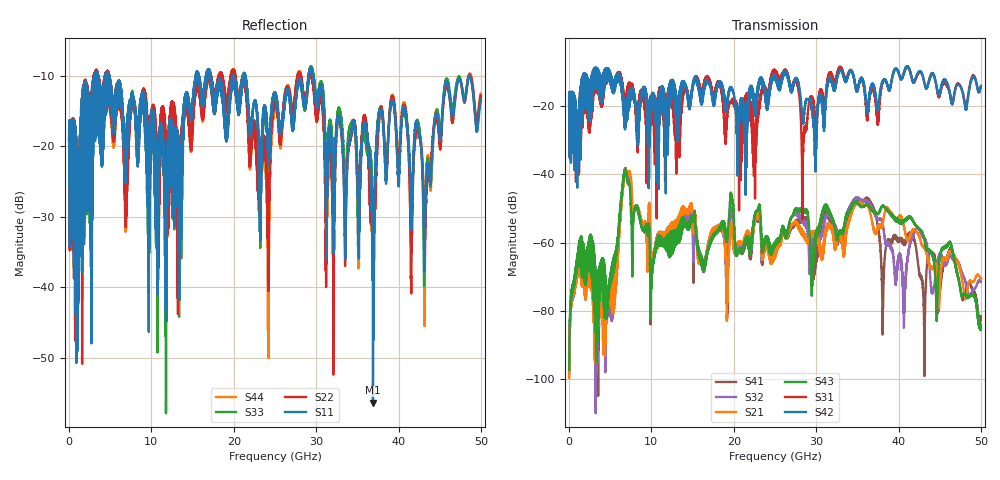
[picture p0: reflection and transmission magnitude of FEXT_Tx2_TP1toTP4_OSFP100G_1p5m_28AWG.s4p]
! Touchstone data
! Created: 27-Feb-2019 by IdEM 12 (12.1.0)
! COMMENTS
!  Created Wed Feb 27 09:43:39 2019
!  64 Port Network Data from SP1.SP block
!  freq  magS1_1  angS1_1  magS1_2  angS1_2  magS1_3  angS1_3  magS1_4  angS1_4
!  magS1_5  angS1_5  magS1_6  angS1_6  magS1_7  angS1_7  magS1_8  angS1_8
!  magS1_9  angS1_9  magS1_10  angS1_10  magS1_11  angS1_11  magS1_12  angS1_12
!  magS1_13  angS1_13  magS1_14  angS1_14  magS1_15  angS1_15  magS1_16  angS1_16
!  magS1_17  angS1_17  magS1_18  angS1_18  magS1_19  angS1_19  magS1_20  angS1_20
!  magS1_21  angS1_21  magS1_22  angS1_22  magS1_23  angS1_23  magS1_24  angS1_24
!  magS1_25  angS1_25  magS1_26  angS1_26  magS1_27  angS1_27  magS1_28  angS1_28
!  magS1_29  angS1_29  magS1_30  angS1_30  magS1_31  angS1_31  magS1_32  angS1_32
!  magS1_33  angS1_33  magS1_34  angS1_34  magS1_35  angS1_35  magS1_36  angS1_36
!  magS1_37  angS1_37  magS1_38  angS1_38  magS1_39  angS1_39  magS1_40  angS1_40
!  magS1_41  angS1_41  magS1_42  angS1_42  magS1_43  angS1_43  magS1_44  angS1_44
!  magS1_45  angS1_45  magS1_46  angS1_46  magS1_47  angS1_47  magS1_48  angS1_48
!  magS1_49  angS1_49  magS1_50  angS1_50  magS1_51  angS1_51  magS1_52  angS1_52
!  magS1_53  angS1_53  magS1_54  angS1_54  magS1_55  angS1_55  magS1_56  angS1_56
!  magS1_57  angS1_57  magS1_58  angS1_58  magS1_59  angS1_59  magS1_60  angS1_60
!  magS1_61  angS1_61  magS1_62  angS1_62  magS1_63  angS1_63  magS1_64  angS1_64
!  magS2_1  angS2_1  magS2_2  angS2_2  magS2_3  angS2_3  magS2_4  angS2_4
!  magS2_5  angS2_5  magS2_6  angS2_6  magS2_7  angS2_7  magS2_8  angS2_8
!  magS2_9  angS2_9  magS2_10  angS2_10  magS2_11  angS2_11  magS2_12  angS2_12
!  magS2_13  angS2_13  magS2_14  angS2_14  magS2_15  angS2_15  magS2_16  angS2_16
!  magS2_17  angS2_17  magS2_18  angS2_18  magS2_19  angS2_19  magS2_20  angS2_20
!  magS2_21  angS2_21  magS2_22  angS2_22  magS2_23  angS2_23  magS2_24  angS2_24
!  magS2_25  angS2_25  magS2_26  angS2_26  magS2_27  angS2_27  magS2_28  angS2_28
!  magS2_29  angS2_29  magS2_30  angS2_30  magS2_31  angS2_31  magS2_32  angS2_32
!  magS2_33  angS2_33  magS2_34  angS2_34  magS2_35  angS2_35  magS2_36  angS2_36
!  magS2_37  angS2_37  magS2_38  angS2_38  magS2_39  angS2_39  magS2_40  angS2_40
!  magS2_41  angS2_41  magS2_42  angS2_42  magS2_43  angS2_43  magS2_44  angS2_44
!  magS2_45  angS2_45  magS2_46  angS2_46  magS2_47  angS2_47  magS2_48  angS2_48
!  magS2_49  angS2_49  magS2_50  angS2_50  magS2_51  angS2_51  magS2_52  angS2_52
!  magS2_53  angS2_53  magS2_54  angS2_54  magS2_55  angS2_55  magS2_56  angS2_56
!  magS2_57  angS2_57  magS2_58  angS2_58  magS2_59  angS2_59  magS2_60  angS2_60
!  magS2_61  angS2_61  magS2_62  angS2_62  magS2_63  angS2_63  magS2_64  angS2_64
!  magS3_1  angS3_1  magS3_2  angS3_2  magS3_3  angS3_3  magS3_4  angS3_4
!  magS3_5  angS3_5  magS3_6  angS3_6  magS3_7  angS3_7  magS3_8  angS3_8
!  magS3_9  angS3_9  magS3_10  angS3_10  magS3_11  angS3_11  magS3_12  angS3_12
!  magS3_13  angS3_13  magS3_14  angS3_14  magS3_15  angS3_15  magS3_16  angS3_16
!  magS3_17  angS3_17  magS3_18  angS3_18  magS3_19  angS3_19  magS3_20  angS3_20
!  magS3_21  angS3_21  magS3_22  angS3_22  magS3_23  angS3_23  magS3_24  angS3_24
!  magS3_25  angS3_25  magS3_26  angS3_26  magS3_27  angS3_27  magS3_28  angS3_28
!  magS3_29  angS3_29  magS3_30  angS3_30  magS3_31  angS3_31  magS3_32  angS3_32
!  magS3_33  angS3_33  magS3_34  angS3_34  magS3_35  angS3_35  magS3_36  angS3_36
!  magS3_37  angS3_37  magS3_38  angS3_38  magS3_39  angS3_39  magS3_40  angS3_40
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# Hz S MA R 50
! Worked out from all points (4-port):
!   5000 points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, 10 MHz to 50 GHz, reference 50 ohm
!   strongest paths, dB at 10 MHz, 12.51 GHz, 25.01 GHz, 37.51 GHz, 50 GHz:
!     S42: -19.6, -13.9, -11.7, -21.0, -14.0
!     S31: -19.6, -16.6, -9.8, -25.4, -14.2
!     S43: -97.3, -60.1, -60.1, -51.6, -84.4
!     S21: -99.7, -56.9, -63.1, -55.3, -70.6
!     S32: -98.0, -58.4, -61.9, -53.1, -71.5
!     S41: -99.1, -58.3, -61.6, -55.7, -81.6
!   lowest |S11| = -56.3 dB at 36.9 GHz (marker M1), VSWR 1.00, Z = 50.1 + j0.121 ohm
!   |S11| at or under -10 dB: 4.861 GHz to 15.4 GHz (10.54 GHz wide, 104 % of centre); 21.38 GHz to 29.07 GHz (7.682 GHz wide, 30.5 % of centre); 29.66 GHz to end of sweep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
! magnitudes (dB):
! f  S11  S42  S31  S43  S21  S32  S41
! 10 MHz  -19.1  -19.6  -19.6  -97.3  -99.7  -98.0  -99.1
! 5.43 GHz  -18.3  -16.2  -15.3  -68.3  -80.3  -78.3  -71.1
! 6.99 GHz  -18.9  -20.6  -18.2  -40.1  -39.1  -39.4  -39.6
! 10.07 GHz  -18.3  -19.4  -20.9  -68.0  -63.8  -64.8  -64.6
! 29.37 GHz  -8.8  -19.5  -17.4  -67.9  -58.0  -64.0  -63.7
! 36.9 GHz  -56.3  -13.6  -14.9  -50.8  -55.2  -50.8  -49.4
! 50 GHz  -13.4  -14.0  -14.2  -84.4  -70.6  -71.5  -81.6
